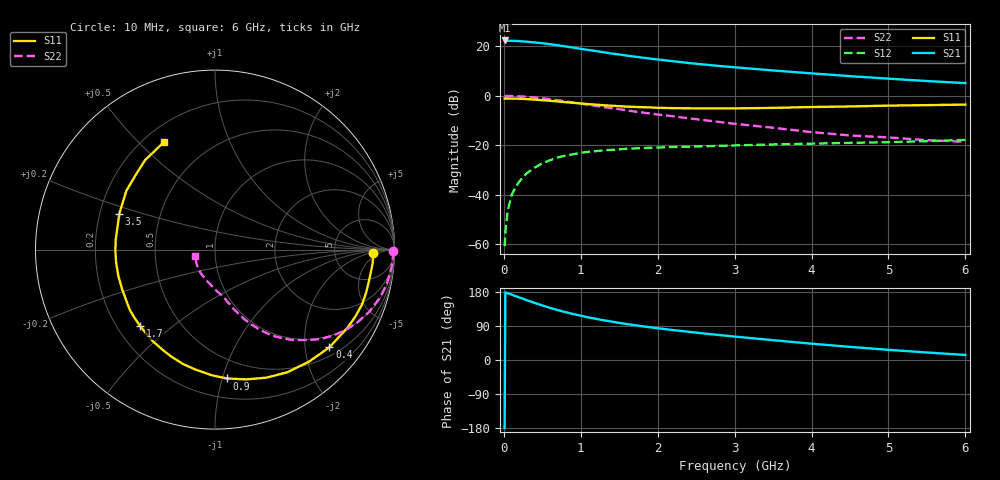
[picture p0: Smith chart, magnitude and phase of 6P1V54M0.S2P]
! Infineon Technologies  Discrete & RF Semiconductors
! BFP540
! Si NPN RF SIEGET Grounded Emitter Transistor in SOT343
! VCE = 1.5 V  IC = 4 mA
! Common Emitter S-Parameters:  April  1999
# GHz  S  MA  R  50
!  f  S11  S21  S12  S22
! GHz  MAG  ANG  MAG  ANG  MAG  ANG  MAG  ANG
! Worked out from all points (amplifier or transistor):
!   36 points, 10 MHz to 6 GHz, reference 50 ohm
!   highest |S21| = 22.4 dB at 10 MHz (marker M1)
!   |S21| within 3 dB of that: start of sweep to 920.2 MHz
!   unconditionally stable (mu >= 1): 3.561 GHz to end of sweep
!   at 250 MHz: K = 0.05, MSG = 27.5 dB, |S12| = -33.0 dB
!   at 1.4 GHz: K = 0.40, MSG = 19.5 dB, |S12| = -21.9 dB
!   at 6 GHz: K = 1.28, MAG = 8.3 dB, |S12| = -17.8 dB
!   lowest NFmin = 0.65 dB at 900 MHz
!   S11 on the Smith chart (normalised r, x): 10 MHz: 16, -2; 400 MHz: 0.69, -2.54; 900 MHz: 0.35, -1.04; 1.7 GHz: 0.29, -0.39; 3.5 GHz: 0.28, +0.17; 6 GHz: 0.28, +0.60
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0.01  0.8819 -1.1  13.22 -179.8  0.0009 70.8  0.9905 -0.5
0.02  0.8821 -2.1  13.07 178.6  0.0017 100.7  0.9972 -1.3
0.05  0.8814 -5.1  13.02 176.2  0.0047 89.3  0.9909 -2.8
0.1  0.8761 -10.3  12.97 172.8  0.0096 87.0  0.9887 -5.6
0.2  0.8744 -20.6  12.81 165.1  0.0183 80.7  0.976 -11.2
0.3  0.8568 -30.6  12.49 157.8  0.0272 76.0  0.9545 -16.7
0.4  0.8383 -40.5  12.04 150.7  0.035 69.9  0.9272 -21.9
0.5  0.815 -50.0  11.64 144.0  0.043 66.0  0.8921 -26.9
0.6  0.7933 -59.5  11.1 137.5  0.0496 62.0  0.8545 -31.7
0.8  0.7434 -76.6  10.04 126.3  0.0614 53.8  0.7749 -39.9
0.9  0.721 -84.7  9.47 121.4  0.0654 50.3  0.7315 -43.5
1.1  0.6769 -99.4  8.49 112.3  0.0736 44.4  0.6595 -49.7
1.4  0.6295 -117.8  7.18 101.5  0.0804 37.5  0.5619 -57.2
1.6  0.6033 -130.0  6.514 94.7  0.085 33.9  0.507 -61.1
1.7  0.5962 -134.5  6.223 92.1  0.086 32.6  0.4798 -62.9
1.9  0.5821 -144.3  5.672 86.4  0.0888 29.8  0.4372 -65.9
2.2  0.5627 -156.8  5.016 79.0  0.092 27.2  0.3849 -69.4
2.8  0.5551 -179.1  4.021 65.9  0.097 23.0  0.2952 -77.0
3.5  0.5693 159.5  3.261 52.3  0.1037 19.8  0.2253 -89.0
4.5  0.6086 136.0  2.501 34.6  0.1115 15.8  0.1575 -117.9
5.5  0.6469 120.4  1.992 19.8  0.1205 14.0  0.1265 -145.4
6  0.6646 115.1  1.81 13.3  0.1283 13.0  0.1171 -162.1
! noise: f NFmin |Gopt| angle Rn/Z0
0.9  0.65  0  0  0
1.8  0.92  0  0  0
2.4  1.12  0  0  0
3  1.25  0  0  0
4  1.42  0  0  0
5  1.88  0  0  0
6  2.15  0  0  0
